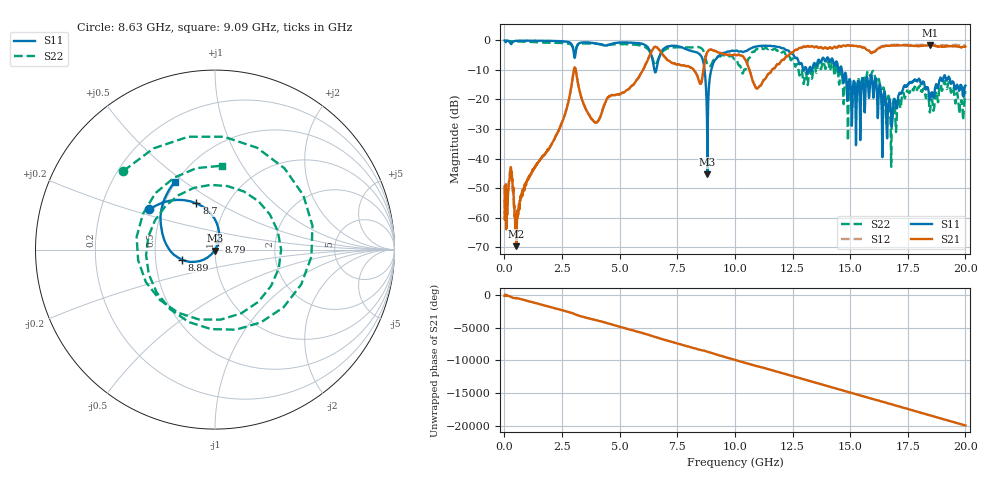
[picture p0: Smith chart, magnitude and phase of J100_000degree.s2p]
!Keysight Technologies,N5222A,MY51421036,A.10.65.16
!Date: Friday, March 31, 2023 14:44:16
!Correction: S11(Full 2 Port(1,2))
!S21(Full 2 Port(1,2))
!S12(Full 2 Port(1,2))
!S22(Full 2 Port(1,2))
!S2P File: Measurements: S11, S21, S12, S22:
# Hz S  dB  R 50
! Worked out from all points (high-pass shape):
!   2000 points, 10 MHz to 20 GHz, reference 50 ohm
!   highest |S21| = -1.65 dB at 18.45 GHz (marker M1); lowest = -69.7 dB at 520 MHz (marker M2)
!   |S21| within 3 dB of the highest: 8.768 GHz to 9.488 GHz (720.1 MHz wide, 7.89 % of centre); 12.37 GHz to end of sweep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
!   lowest |S11| = -45.4 dB at 8.81 GHz (marker M3), VSWR 1.01, Z = 49.8 - j0.502 ohm
!   |S11| at or under -10 dB: 6.507 GHz to 6.591 GHz (83.13 MHz wide, 1.27 % of centre); 8.684 GHz to 8.977 GHz (292.7 MHz wide, 3.32 % of centre); 14.64 GHz to end of sweep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
!   |S22| runs from -42.8 to -0.1 dB; largest |S21 - S12| = 0.063
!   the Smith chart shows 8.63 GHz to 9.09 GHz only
!   S11 on the Smith chart (normalised r, x): 8.63 GHz: 0.43, +0.23; 8.7 GHz: 0.72, +0.40; 8.79 GHz: 1.04, +0.09; 8.89 GHz: 0.68, -0.08; 9.09 GHz: 0.49, +0.46
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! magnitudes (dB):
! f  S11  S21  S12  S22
! 10 MHz  0.0  -49.6  -53.8  -0.1
! 280 MHz  -1.2  -42.9  -43.3  -0.3
! 520 MHz  -0.2  -69.7  -64.1  -0.3
! 3.03 GHz  -5.3  -9.4  -9.4  -3.7
! 3.35 GHz  -0.8  -19.7  -19.7  -1.1
! 4.02 GHz  -1.1  -27.7  -27.6  -1.2
! 6.68 GHz  -6.6  -2.9  -2.8  -6.3
! 8.63 GHz  -7.4  -10.4  -10.4  -3.4
! 8.7 GHz  -11.1  -7.0  -6.9  -5.1
! 8.79 GHz  -26.8  -4.2  -4.2  -7.9
! 8.81 GHz  -45.4  -3.9  -3.9  -8.3
! 8.89 GHz  -14.2  -3.2  -3.2  -8.8
! 9.09 GHz  -7.2  -3.5  -3.5  -6.6
! 10.01 GHz  -3.6  -4.9  -4.9  -6.3
! 10.99 GHz  -2.0  -16.2  -16.2  -3.0
! 13.34 GHz  -10.3  -1.9  -1.9  -13.0
! 14.32 GHz  -8.6  -2.2  -2.1  -12.0
! 14.99 GHz  -13.2  -1.9  -1.7  -13.9
! 15.98 GHz  -16.4  -4.1  -3.9  -10.4
! 16.67 GHz  -21.0  -1.8  -1.6  -18.8
! 18.45 GHz  -20.1  -1.7  -1.4  -24.2
! 20 GHz  -15.3  -2.1  -1.6  -17.2
